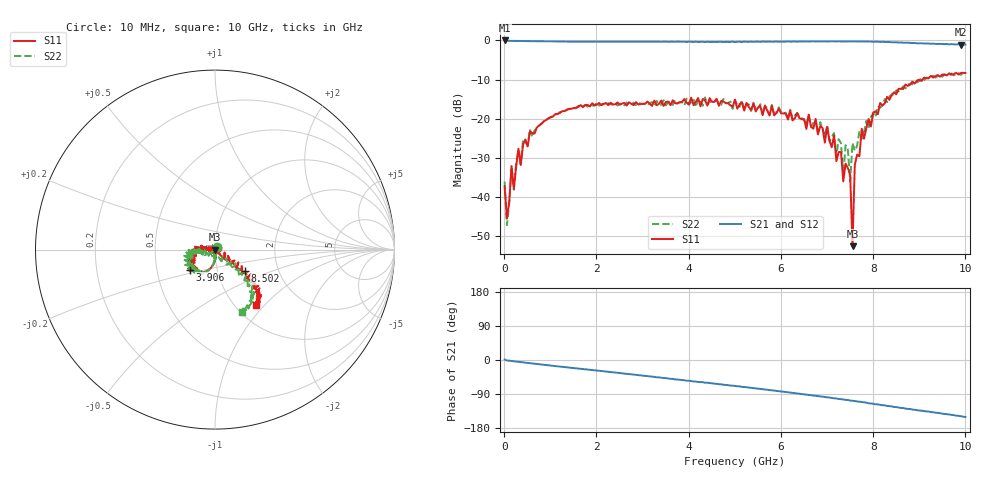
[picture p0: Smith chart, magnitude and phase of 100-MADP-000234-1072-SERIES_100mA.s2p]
!Agilent Technologies,E8364C,MY48140145,A.09.42.15
!Agilent E8364C: A.09.42.15
!Date: Wednesday, December 02, 2020 08:33:13
!Correction: S11(Full 2 Port(1,2))
!S21(Full 2 Port(1,2))
!S12(Full 2 Port(1,2))
!S22(Full 2 Port(1,2))
!S2P File: Measurements: S11, S21, S12, S22:
# Hz S  dB  R 50
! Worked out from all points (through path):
!   201 points, 10 MHz to 10 GHz, reference 50 ohm
!   highest |S21| = -0.01 dB at 10 MHz (marker M1); lowest = -1.1 dB at 9.9 GHz (marker M2)
!   group delay of S21, straight-line fit = 41 ps
!   lowest |S11| = -52.5 dB at 7.552 GHz (marker M3), VSWR 1.00, Z = 49.8 - j0.0734 ohm
!   |S11| at or under -10 dB: start of sweep to 9.071 GHz
!   |S22| runs from -47.1 to -8.2 dB; largest |S21 - S12| = 0.022
!   S11 on the Smith chart (normalised r, x): 10 MHz: 1.02, +0.02; 3.906 GHz: 0.74, -0.17; 8.502 GHz: 1.35, -0.34; 10 GHz: 1.24, -0.89
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1e7  -37.29 46.9  -0.01 1.0  -0.06 -0.3  -36.03 49.1
5.995e7  -45.37 -72.4  -0.10 -1.0  -0.09 -1.1  -47.14 -76.1
1.5985e8  -32.05 -79.4  -0.12 -2.7  -0.10 -2.7  -32.32 -76.2
2.098e8  -37.91 -70.2  -0.12 -3.5  -0.12 -3.4  -38.09 -80.1
3.097e8  -27.62 -86.4  -0.15 -4.9  -0.15 -4.9  -27.97 -82.7
5.5945e8  -23.22 -93.9  -0.20 -8.5  -0.18 -8.5  -22.68 -90.9
1.7083e9  -17.04 -119.1  -0.31 -24.1  -0.29 -23.8  -16.84 -117.7
3.35665e9  -16.17 -137.8  -0.30 -45.9  -0.32 -46.1  -16.27 -127.6
3.9061e9  -14.95 -140.5  -0.34 -53.3  -0.35 -53.9  -16.57 -135.9
5.005e9  -15.13 -151.1  -0.42 -68.7  -0.39 -68.5  -15.13 -168.5
6.7033e9  -22.52 171.6  -0.24 -93.8  -0.21 -93.6  -21.00 174.9
7.15285e9  -24.24 166.3  -0.27 -100.9  -0.28 -101.3  -23.64 -151.7
7.35265e9  -35.98 -102.2  -0.26 -104.3  -0.23 -103.9  -34.34 -144.1
7.4026e9  -31.44 146.9  -0.24 -105.1  -0.24 -105.1  -26.74 -138.6
7.5025e9  -34.35 -44.7  -0.26 -107.1  -0.23 -106.5  -36.02 -115.2
7.55245e9  -52.50 -161.9  -0.25 -107.6  -0.25 -107.9  -26.17 -95.8
7.6024e9  -31.72 -45.7  -0.26 -108.5  -0.24 -108.5  -28.16 -72.6
7.75225e9  -22.54 -44.0  -0.29 -111.2  -0.24 -110.9  -25.07 -37.7
8.35165e9  -15.16 -31.5  -0.41 -121.9  -0.44 -121.9  -14.31 -46.3
8.5015e9  -13.74 -36.0  -0.47 -124.3  -0.50 -124.7  -12.71 -44.5
9.9001e9  -8.31 -54.1  -1.07 -148.4  -0.99 -148.2  -8.79 -64.5
1e10  -8.33 -53.2  -1.06 -150.2  -1.05 -150.3  -8.44 -66.7
